| TEXAS INSTRUMENTS INCORPORATED
| Standard Linear and Logic Group
| IBIS Model of SN74CBT16210C
| 20-BIT FET BUS SWITCH WITH -2 V UNDERSHOOT-PROTECTION
| This file contains package information for the following:
|  TSSOP 48-pin (DGG) package as [Component] CBT16210C_DGG
|  TVSOP 48-pin (DGV) package as [Component] CBT16210C_DGV
|  SSOP 48-pin (DL) package as [Component] CBT16210C_DL
| This device can be powered at the following Vccs:
|  5 volt Vcc
|  4 volt Vcc
| This file provides unique models under the [Model Selector] for each Vcc.
| For operation at a specific Vcc, select the appropriate model after each
| [Model Selector] keyword.
[IBIS Ver]   3.2
[Comment char]  |_char
[File Name]   sn74cbt16210c.ibs
[File Rev]   1.1 | a_die
[Date]   June 24, 2003
[Source]   Data created from TI-SPICE simulations at TI-SLL.
[Notes]   The following is an IBIS list for the SN74CBT16210C.
   Please contact sllibis@ti.com with questions and
   comments concerning SLL IBIS models.
   - Non-monotonic data due to FET characteristics.
   - C_comp values are taken at a different test condition than
   the Cio in data sheet.
   - Power-clamp data has been deleted since there is no
   power-clamp diode in the device.
[Disclaimer] Property of Texas Instruments Incorporated. Unauthorized
   reproduction and/or distribution is strictly prohibited.
   This product is protected under copyright law.
   Created 2003,(C) Copyright 2003, Texas Instruments
   Incorporated, All Rights Reserved
   UNLESS THERE IS A SIGNED, WRITTEN AGREEMENT TO THE
   CONTRARY, TEXAS INSTRUMENTS (TI) IS PROVIDING THE IBIS
   MODELS AND WITHOUT ANY WARRANTY, EXPRESSED OR
   IMPLIED. TI assumes no liability for:
   1) the accuracy of the IBIS models provided to your
   company;
   2) the proper functioning of these IBIS Models in your
   design or for any resulting applications; or
   3) infringement of patents, copyrights or intellectual
   property rights resulting from your use of these IBIS
   models.
   TI provides IBIS Models as a service to our customers.
   You and your company shall not distribute, sell or give
   these models to anyone else without prior written
   permission from TI.
   TI reserves the right to make changes to our products or
   to discontinue any semiconductor product or service
   without notice, and advises our customers to obtain the
   latest version of relevant information to verify, before
   placing orders, that the information being relied on is
   current.
   Please be aware that your receipt and use of the IBIS
   information provided shall serve as acceptance of these
   terms and conditions. If you do not accept these terms,
   you should return or destroy the IBIS models and any
   other accompanying information immediately.
| Component CBT16210C_DGG 48-pin TSSOP
[Component]   CBT16210C_DGG
[Manufacturer]   Texas Instruments, Inc.
[Package]
|   typ   min   max
R_pkg   5.400e-02   4.000e-02   8.300e-02
L_pkg   3.546e-09   2.838e-09   5.045e-09
C_pkg   5.580e-13   4.120e-13   7.380e-13
[Pin]   signal_name   model_name   R_pin   L_pin   C_pin
1   NC   NC   7.600e-02   5.003e-09   7.120e-13
2   1A1   CBT16210C_IO   7.600e-02   4.539e-09   7.230e-13
3   1A2   CBT16210C_IO   8.300e-02   4.357e-09   7.080e-13
4   1A3   CBT16210C_IO   4.200e-02   3.999e-09   6.830e-13
5   1A4   CBT16210C_IO   4.200e-02   3.806e-09   6.700e-13
6   1A5   CBT16210C_IO   4.300e-02   3.603e-09   6.160e-13
7   1A6   CBT16210C_IO   4.400e-02   3.440e-09   5.520e-13
8   GND   GND   4.600e-02   3.306e-09   5.090e-13
9   1A7   CBT16210C_IO   4.700e-02   3.194e-09   4.820e-13
10   1A8   CBT16210C_IO   4.800e-02   3.088e-09   4.630e-13
11   1A9   CBT16210C_IO   5.000e-02   2.987e-09   4.350e-13
12   1A10   CBT16210C_IO   5.100e-02   2.910e-09   4.230e-13
13   2A1   CBT16210C_IO   5.300e-02   2.850e-09   4.230e-13
14   2A2   CBT16210C_IO   5.200e-02   2.886e-09   4.210e-13
15   VCC   POWER   5.100e-02   2.883e-09   4.190e-13
16   2A3   CBT16210C_IO   5.000e-02   2.941e-09   4.300e-13
17   GND   GND   4.900e-02   3.031e-09   4.570e-13
18   2A4   CBT16210C_IO   4.700e-02   3.131e-09   4.760e-13
19   2A5   CBT16210C_IO   4.600e-02   3.244e-09   5.030e-13
20   2A6   CBT16210C_IO   4.400e-02   3.387e-09   5.500e-13
21   2A7   CBT16210C_IO   4.300e-02   3.566e-09   6.320e-13
22   2A8   CBT16210C_IO   4.200e-02   3.801e-09   6.870e-13
23   2A9   CBT16210C_IO   4.100e-02   3.961e-09   6.870e-13
24   2A10   CBT16210C_IO   8.100e-02   4.291e-09   7.110e-13
25   2B10   CBT16210C_IO   8.300e-02   4.336e-09   7.080e-13
26   2B9   CBT16210C_IO   4.000e-02   3.957e-09   6.840e-13
27   2B8   CBT16210C_IO   4.200e-02   3.789e-09   6.800e-13
28   2B7   CBT16210C_IO   4.300e-02   3.540e-09   6.240e-13
29   2B6   CBT16210C_IO   4.400e-02   3.361e-09   5.460e-13
30   2B5   CBT16210C_IO   4.600e-02   3.222e-09   4.980e-13
31   2B4   CBT16210C_IO   4.700e-02   3.110e-09   4.710e-13
32   GND   GND   4.800e-02   3.012e-09   4.510e-13
33   2B3   CBT16210C_IO   5.000e-02   2.934e-09   4.230e-13
34   2B2   CBT16210C_IO   5.100e-02   2.879e-09   4.120e-13
35   2B1   CBT16210C_IO   5.200e-02   2.883e-09   4.130e-13
36   1B10   CBT16210C_IO   5.200e-02   2.887e-09   4.160e-13
37   1B9   CBT16210C_IO   5.100e-02   2.897e-09   4.160e-13
38   1B8   CBT16210C_IO   5.000e-02   2.965e-09   4.270e-13
39   1B7   CBT16210C_IO   4.800e-02   3.047e-09   4.550e-13
40   1B6   CBT16210C_IO   4.700e-02   3.138e-09   4.740e-13
41   GND   GND   4.600e-02   3.250e-09   5.030e-13
42   1B5   CBT16210C_IO   4.400e-02   3.390e-09   5.500e-13
43   1B4   CBT16210C_IO   4.300e-02   3.546e-09   6.260e-13
44   1B3   CBT16210C_IO   4.200e-02   3.783e-09   6.860e-13
45   1B2   CBT16210C_IO   4.000e-02   3.955e-09   6.820e-13
46   1B1   CBT16210C_IO   8.300e-02   4.330e-09   7.010e-13
47   2NOE   CBT16210C_IN   7.700e-02   4.562e-09   7.240e-13
48   1NOE   CBT16210C_IN   7.500e-02   5.029e-09   7.120e-13
| Component CBT16210C_DGV 48-pin TVSOP
[Component]   CBT16210C_DGV
[Manufacturer]   Texas Instruments, Inc.
[Package]
|   typ   min   max
R_pkg   6.300e-02   5.000e-02   8.400e-02
L_pkg   2.945e-09   2.394e-09   3.939e-09
C_pkg   3.910e-13   2.710e-13   5.880e-13
[Pin]   signal_name   model_name   R_pin   L_pin   C_pin
1   NC   NC   6.800e-02   3.933e-09   5.880e-13
2   1A1   CBT16210C_IO   6.800e-02   3.568e-09   5.870e-13
3   1A2   CBT16210C_IO   7.600e-02   3.464e-09   5.150e-13
4   1A3   CBT16210C_IO   8.400e-02   3.444e-09   4.590e-13
5   1A4   CBT16210C_IO   8.100e-02   3.277e-09   4.270e-13
6   1A5   CBT16210C_IO   7.400e-02   3.136e-09   3.870e-13
7   1A6   CBT16210C_IO   6.900e-02   2.970e-09   4.010e-13
8   GND   GND   5.000e-02   2.785e-09   3.790e-13
9   1A7   CBT16210C_IO   5.100e-02   2.685e-09   3.200e-13
10   1A8   CBT16210C_IO   5.300e-02   2.611e-09   3.160e-13
11   1A9   CBT16210C_IO   5.300e-02   2.495e-09   2.970e-13
12   1A10   CBT16210C_IO   5.300e-02   2.435e-09   2.920e-13
13   2A1   CBT16210C_IO   5.500e-02   2.401e-09   2.730e-13
14   2A2   CBT16210C_IO   5.500e-02   2.399e-09   2.840e-13
15   VCC   POWER   5.400e-02   2.406e-09   2.890e-13
16   2A3   CBT16210C_IO   5.300e-02   2.450e-09   2.930e-13
17   GND   GND   5.100e-02   2.544e-09   3.110e-13
18   2A4   CBT16210C_IO   5.100e-02   2.626e-09   3.150e-13
19   2A5   CBT16210C_IO   5.000e-02   2.727e-09   3.690e-13
20   2A6   CBT16210C_IO   6.500e-02   2.903e-09   3.930e-13
21   2A7   CBT16210C_IO   7.500e-02   3.091e-09   3.860e-13
22   2A8   CBT16210C_IO   8.200e-02   3.272e-09   4.280e-13
23   2A9   CBT16210C_IO   8.200e-02   3.393e-09   4.570e-13
24   2A10   CBT16210C_IO   7.300e-02   3.380e-09   5.080e-13
25   2B10   CBT16210C_IO   7.600e-02   3.428e-09   5.170e-13
26   2B9   CBT16210C_IO   8.100e-02   3.395e-09   4.680e-13
27   2B8   CBT16210C_IO   8.000e-02   3.255e-09   4.310e-13
28   2B7   CBT16210C_IO   7.100e-02   3.064e-09   3.860e-13
29   2B6   CBT16210C_IO   6.100e-02   2.878e-09   3.890e-13
30   2B5   CBT16210C_IO   5.000e-02   2.710e-09   3.630e-13
31   2B4   CBT16210C_IO   5.000e-02   2.606e-09   3.110e-13
32   GND   GND   5.200e-02   2.534e-09   3.060e-13
33   2B3   CBT16210C_IO   5.200e-02   2.439e-09   2.890e-13
34   2B2   CBT16210C_IO   5.300e-02   2.399e-09   2.860e-13
35   2B1   CBT16210C_IO   5.500e-02   2.394e-09   2.820e-13
36   1B10   CBT16210C_IO   5.400e-02   2.402e-09   2.830e-13
37   1B9   CBT16210C_IO   5.400e-02   2.423e-09   2.880e-13
38   1B8   CBT16210C_IO   5.300e-02   2.474e-09   2.920e-13
39   1B7   CBT16210C_IO   5.100e-02   2.569e-09   3.090e-13
40   1B6   CBT16210C_IO   5.100e-02   2.638e-09   3.130e-13
41   GND   GND   5.100e-02   2.742e-09   3.660e-13
42   1B5   CBT16210C_IO   6.400e-02   2.917e-09   3.900e-13
43   1B4   CBT16210C_IO   7.400e-02   3.083e-09   3.830e-13
44   1B3   CBT16210C_IO   8.100e-02   3.249e-09   4.300e-13
45   1B2   CBT16210C_IO   8.300e-02   3.400e-09   4.550e-13
46   1B1   CBT16210C_IO   7.500e-02   3.427e-09   5.050e-13
47   2NOE   CBT16210C_IN   7.100e-02   3.585e-09   5.780e-13
48   1NOE   CBT16210C_IN   6.900e-02   3.939e-09   5.810e-13
| Component CBT16210C_DL 48-pin SSOP
[Component]   CBT16210C_DL
[Manufacturer]   Texas Instruments, Inc.
[Package]
|   typ   min   max
R_pkg   5.500e-02   4.800e-02   6.700e-02
L_pkg   6.539e-09   4.803e-09   9.746e-09
C_pkg   8.570e-13   5.000e-13   1.351e-12
[Pin]   signal_name   model_name   R_pin   L_pin   C_pin
1   NC   NC   6.400e-02   9.646e-09   1.202e-12
2   1A1   CBT16210C_IO   5.900e-02   8.723e-09   1.348e-12
3   1A2   CBT16210C_IO   5.900e-02   8.139e-09   1.223e-12
4   1A3   CBT16210C_IO   5.600e-02   7.554e-09   1.088e-12
5   1A4   CBT16210C_IO   5.400e-02   6.991e-09   9.660e-13
6   1A5   CBT16210C_IO   5.300e-02   6.659e-09   9.730e-13
7   1A6   CBT16210C_IO   5.500e-02   6.321e-09   9.050e-13
8   GND   GND   5.600e-02   5.942e-09   7.130e-13
9   1A7   CBT16210C_IO   5.700e-02   5.768e-09   6.780e-13
10   1A8   CBT16210C_IO   5.400e-02   5.459e-09   6.310e-13
11   1A9   CBT16210C_IO   5.100e-02   5.224e-09   6.380e-13
12   1A10   CBT16210C_IO   4.800e-02   5.088e-09   6.010e-13
13   2A1   CBT16210C_IO   5.100e-02   4.803e-09   5.000e-13
14   2A2   CBT16210C_IO   5.000e-02   5.021e-09   5.180e-13
15   VCC   POWER   4.800e-02   5.088e-09   6.010e-13
16   2A3   CBT16210C_IO   5.100e-02   5.224e-09   6.380e-13
17   GND   GND   5.400e-02   5.459e-09   6.310e-13
18   2A4   CBT16210C_IO   5.700e-02   5.768e-09   6.770e-13
19   2A5   CBT16210C_IO   5.500e-02   5.942e-09   7.150e-13
20   2A6   CBT16210C_IO   5.500e-02   6.321e-09   9.070e-13
21   2A7   CBT16210C_IO   5.300e-02   6.659e-09   9.720e-13
22   2A8   CBT16210C_IO   5.400e-02   6.991e-09   9.660e-13
23   2A9   CBT16210C_IO   5.600e-02   7.554e-09   1.087e-12
24   2A10   CBT16210C_IO   5.900e-02   8.139e-09   1.223e-12
25   2B10   CBT16210C_IO   6.000e-02   8.184e-09   1.224e-12
26   2B9   CBT16210C_IO   5.600e-02   7.543e-09   1.087e-12
27   2B8   CBT16210C_IO   5.400e-02   7.005e-09   9.690e-13
28   2B7   CBT16210C_IO   5.600e-02   6.714e-09   9.750e-13
29   2B6   CBT16210C_IO   5.800e-02   6.384e-09   9.090e-13
30   2B5   CBT16210C_IO   5.700e-02   5.976e-09   7.170e-13
31   2B4   CBT16210C_IO   5.700e-02   5.743e-09   6.770e-13
32   GND   GND   5.400e-02   5.468e-09   6.310e-13
33   2B3   CBT16210C_IO   5.500e-02   5.329e-09   6.440e-13
34   2B2   CBT16210C_IO   5.200e-02   5.189e-09   6.060e-13
35   2B1   CBT16210C_IO   5.200e-02   5.053e-09   5.190e-13
36   1B10   CBT16210C_IO   5.200e-02   5.093e-09   5.210e-13
37   1B9   CBT16210C_IO   5.100e-02   5.179e-09   6.080e-13
38   1B8   CBT16210C_IO   5.400e-02   5.314e-09   6.450e-13
39   1B7   CBT16210C_IO   5.500e-02   5.511e-09   6.320e-13
40   1B6   CBT16210C_IO   5.700e-02   5.770e-09   6.770e-13
41   GND   GND   5.600e-02   5.956e-09   7.160e-13
42   1B5   CBT16210C_IO   5.500e-02   6.320e-09   9.050e-13
43   1B4   CBT16210C_IO   5.200e-02   6.621e-09   9.680e-13
44   1B3   CBT16210C_IO   5.300e-02   6.974e-09   9.660e-13
45   1B2   CBT16210C_IO   5.700e-02   7.571e-09   1.089e-12
46   1B1   CBT16210C_IO   5.700e-02   8.097e-09   1.219e-12
47   2NOE   CBT16210C_IN   5.900e-02   8.723e-09   1.349e-12
48   1NOE   CBT16210C_IN   6.100e-02   9.560e-09   1.199e-12
[Series Switch Groups]
| Function Group States
On  1 /   | 1A1-1A10->1B1-1B10 1NOE Low
On  2 /   | 2A1-2A10->2B1-2B10 2NOE Low
On  1 2 /   | ENABLE BOTH
[Series Pin Mapping]   pin_2   model_name   function_table_group
2   46   CBT16210C_IO_50_S   1
| 2   46   CBT16210C_IO_40_S   1
3   45   CBT16210C_IO_50_S   1
| 3   45   CBT16210C_IO_40_S   1
4   44   CBT16210C_IO_50_S   1
| 4   44   CBT16210C_IO_40_S   1
5   43   CBT16210C_IO_50_S   1
| 5   43   CBT16210C_IO_40_S   1
6   42   CBT16210C_IO_50_S   1
| 6   42   CBT16210C_IO_40_S   1
7   40   CBT16210C_IO_50_S   1
| 7   40   CBT16210C_IO_40_S   1
9   39   CBT16210C_IO_50_S   1
| 9   39   CBT16210C_IO_40_S   1
10   38   CBT16210C_IO_50_S   1
| 10   38   CBT16210C_IO_40_S   1
11   37   CBT16210C_IO_50_S   1
| 11   37   CBT16210C_IO_40_S   1
12   36   CBT16210C_IO_50_S   1
| 12   36   CBT16210C_IO_40_S   1
13   35   CBT16210C_IO_50_S   2
| 13   35   CBT16210C_IO_40_S   2
14   34   CBT16210C_IO_50_S   2
| 14   34   CBT16210C_IO_40_S   2
16   33   CBT16210C_IO_50_S   2
| 16   33   CBT16210C_IO_40_S   2
18   31   CBT16210C_IO_50_S   2
| 18   31   CBT16210C_IO_40_S   2
19   30   CBT16210C_IO_50_S   2
| 19   30   CBT16210C_IO_40_S   2
20   29   CBT16210C_IO_50_S   2
| 20   29   CBT16210C_IO_40_S   2
21   28   CBT16210C_IO_50_S   2
| 21   28   CBT16210C_IO_40_S   2
22   27   CBT16210C_IO_50_S   2
| 22   27   CBT16210C_IO_40_S   2
23   26   CBT16210C_IO_50_S   2
| 23   26   CBT16210C_IO_40_S   2
24   25   CBT16210C_IO_50_S   2
| 24   25   CBT16210C_IO_40_S   2
| Model CBT16210C_IN
[Model Selector]   CBT16210C_IN
CBT16210C_IN_50   5 volt Vcc
CBT16210C_IN_40   4 volt Vcc
| Model CBT16210C_IO
[Model Selector]   CBT16210C_IO
CBT16210C_IO_50   5 volt Vcc
CBT16210C_IO_40   4 volt Vcc
| Model CBT16210C_IO_S
[Model Selector]   CBT16210C_IO_S
CBT16210C_IO_50_S   5 volt Vcc
CBT16210C_IO_40_S   4 volt Vcc
[Model]   CBT16210C_IO_50_S
Model_type  Series_switch
| variable   typ   min   max
C_comp   0   0   0
[Temperature Range]   40   100   -40
| Ambient temperature   25   85   -40
[Voltage range]   5   4.5   5.5
[On]
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[Off]
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[Model]   CBT16210C_IO_40_S
Model_type  Series_switch
| variable   typ   min   max
C_comp   0   0   0
[Temperature Range]   40   100   -40
| Ambient temperature   25   85   -40
[Voltage range]   4   4   4
[On]
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[Off]
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| Models and submodels in the file (6): CBT16210C_IN_50 (Input), CBT16210C_IN_40 (Input), CBT16210C_IO_50_S (Series_switch), CBT16210C_IO_50 (Terminator), CBT16210C_IO_40_S (Series_switch), CBT16210C_IO_40 (Terminator)
